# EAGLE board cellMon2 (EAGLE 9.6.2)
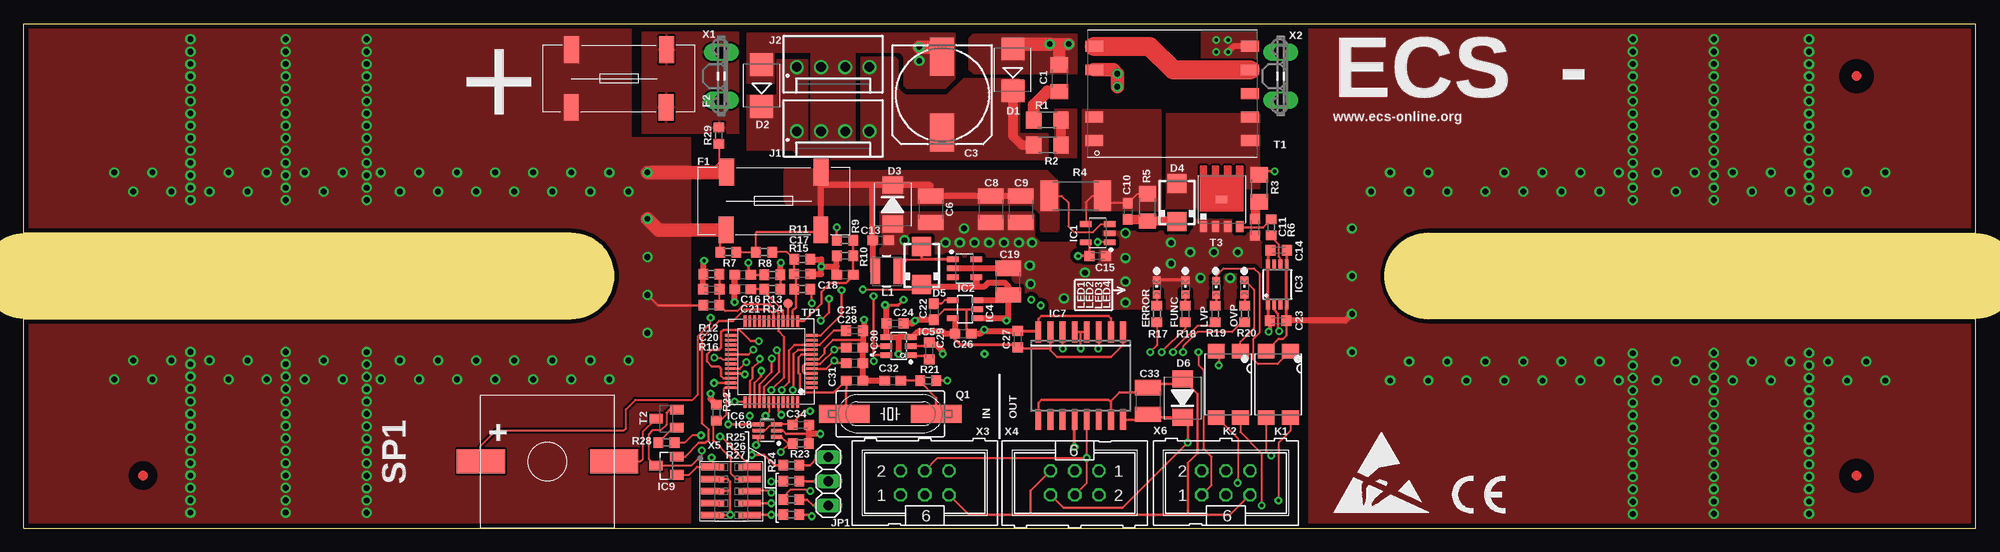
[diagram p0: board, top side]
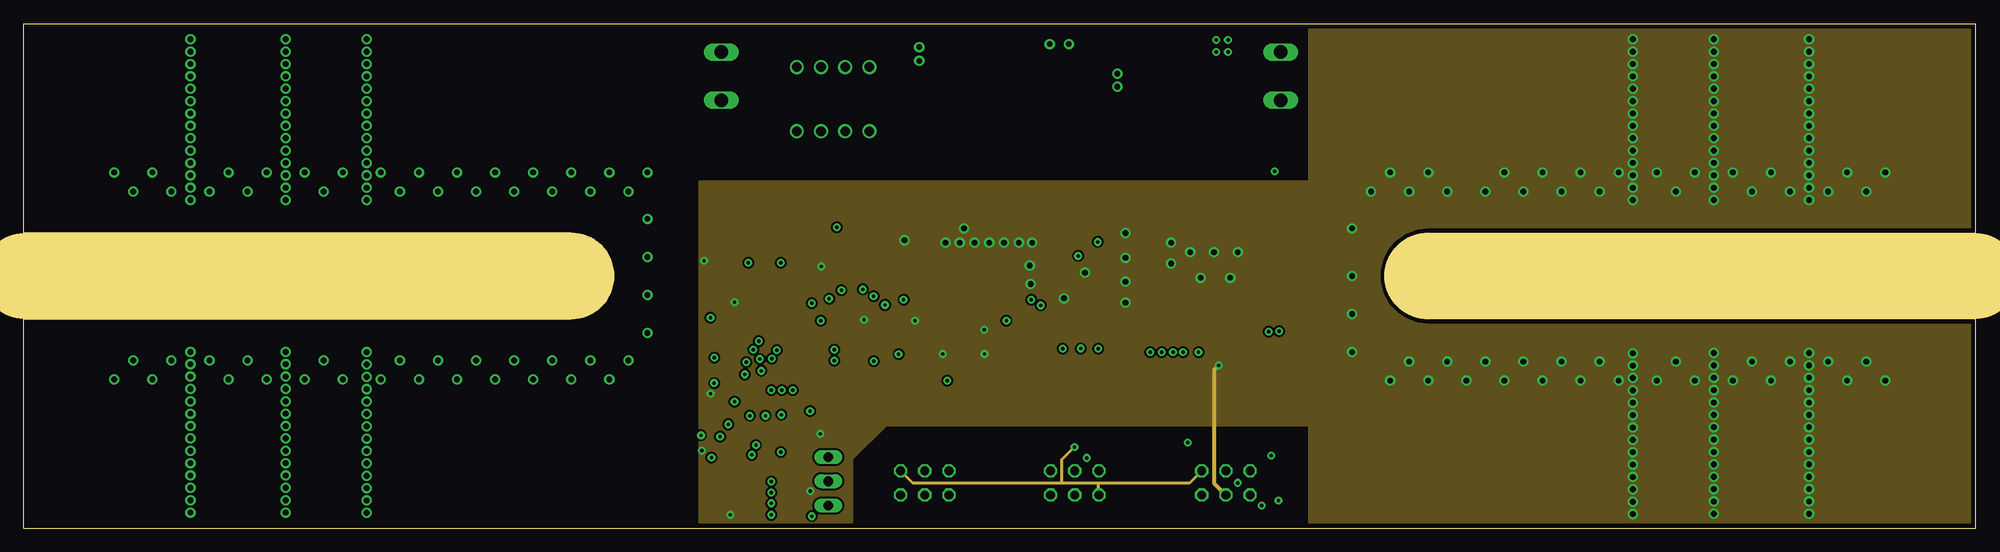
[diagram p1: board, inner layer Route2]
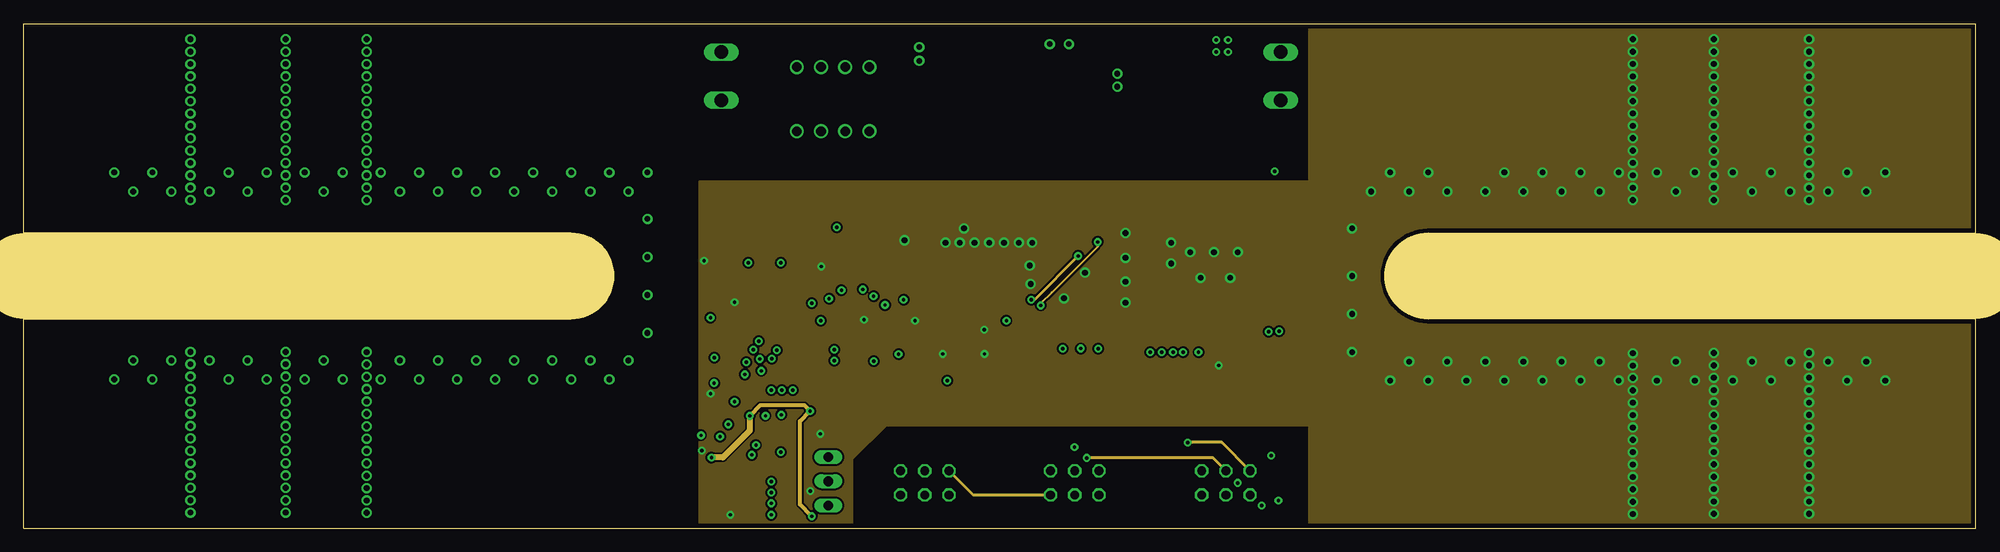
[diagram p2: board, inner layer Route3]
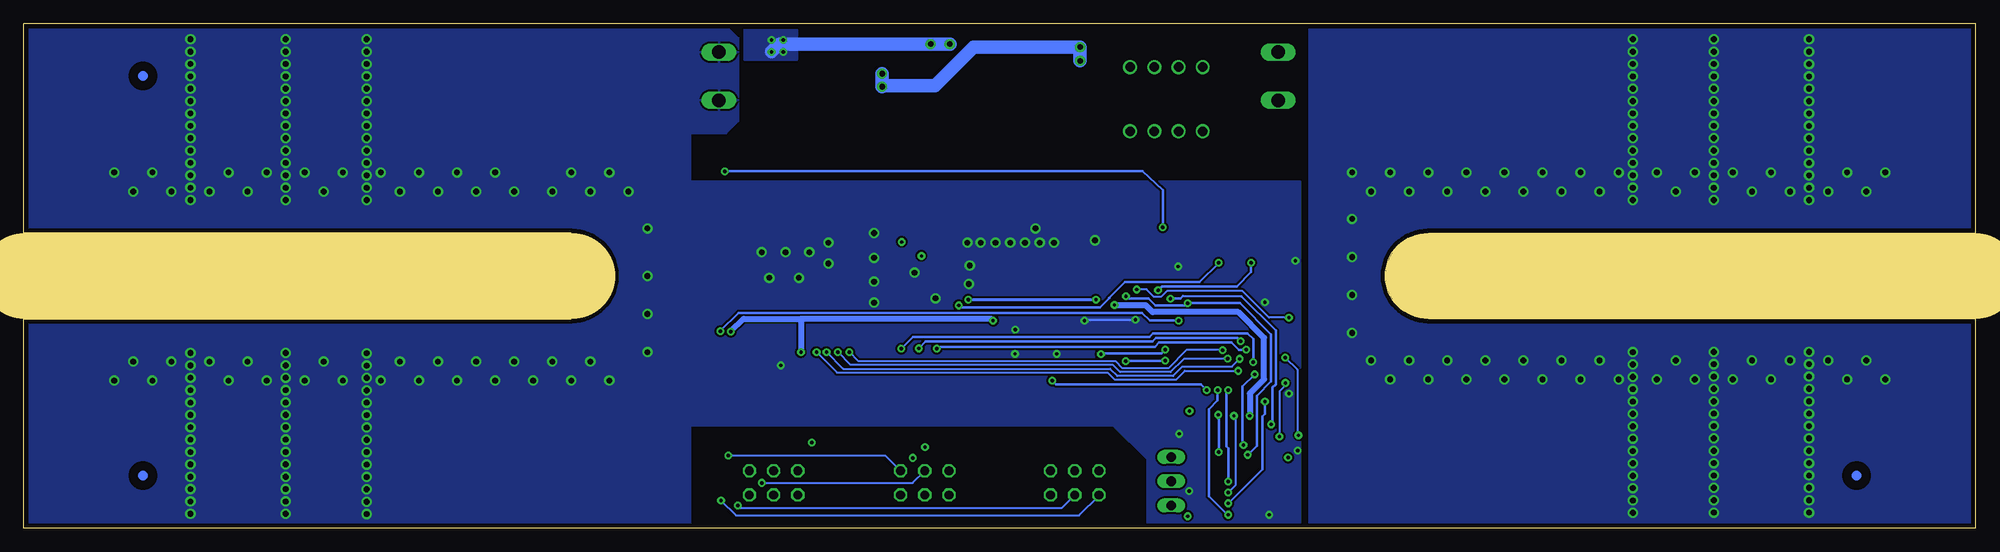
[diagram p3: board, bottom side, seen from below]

Size 205 x 53 mm. Coordinates in mm from the lower left corner, seen from the top.
Outline: 0,0 205,0 205,22 147.5,22 arc-180 147.5,31 205,31 205,53 0,53 0,31 57.5,31 arc-180 57.5,22 0,22 0,0
Copper layers (1+2*3+16): Top 0.018mm / dielectric 0.36mm / Route2 0.035mm / dielectric 0.71mm / Route3 0.035mm / dielectric 0.36mm / Bottom 0.018mm
Design rules "multi-cb_070um-cu *": minimum track width 8mil, minimum drill 12mil, track to track 8mil, track to pad 8mil, pad to pad 8mil, via to via 8mil, smd to smd 8mil, copper to edge 20mil, drill to drill 8mil, minimum pad ring 9mil, minimum via ring 9mil, stop-mask expansion 3mil, vias tented up to drill 0mil, thermal gap 8mil
Milling: 2 lines

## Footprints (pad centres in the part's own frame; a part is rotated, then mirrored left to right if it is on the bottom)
C1206 = smd 1.6 x 1.8: 1 -1.4,0; 2 1.4,0
153CLV-1010 = smd 4 x 2.5: + 4,0; - -4,0
C1210 = smd 1.6 x 2.7: 1 -1.4,0; 2 1.4,0
C0603 = smd 1.1 x 1: 1 -0.85,0; 2 0.85,0
C0603K = smd 1.05 x 1.08: 1 -0.875,0; 2 0.875,0
SMB = smd 2.4 x 2.4: A 2.2,0; C -2.2,0
SMBJ = smd 1.78 x 2.16: A 2.04,0; C -2.03,0
SMA = smd 2 x 2: A 2,0; C -2,0
3588 = smd 1.57 x 2.82: 1A -4.955,3.03; 1B -4.995,-3.03; 2A 4.995,3.03; 2B 4.955,-3.03
SOT95P280X110-5N = smd 1.209 x 0.589: 1 -1.253,0.95; 2 -1.253,0; 3 -1.253,-0.95; 4 1.253,-0.95; 5 1.253,0.95
MSOP8 = smd 0.4 x 1.2: 1 -0.975,-2.05; 2 -0.325,-2.05; 3 0.325,-2.05; 4 0.975,-2.05; 5 0.975,2.05; 6 0.325,2.05; 7 -0.325,2.05; 8 -0.975,2.05
SOT25 = smd 0.55 x 1.2: 1 -0.95,-1.3; 2 0,-1.3; 3 0.95,-1.3; 4 0.95,1.3; 5 -0.95,1.3
SOT23-6 = smd 0.55 x 1.2: 1 -0.95,-1.3; 2 0,-1.3; 3 0.95,-1.3; 4 0.95,1.3; 5 0,1.3; 6 -0.95,1.3
LQFP48 = smd 0.29 x 1.2: 1 -2.75,-4.25; 2 -2.25,-4.25; 3 -1.75,-4.25; 4 -1.25,-4.25; 5 -0.75,-4.25; 6 -0.25,-4.25; 7 0.25,-4.25; 8 0.75,-4.25; 9 1.25,-4.25; 10 1.75,-4.25; 11 2.25,-4.25; 12 2.75,-4.25; 25 2.75,4.25; 26 2.25,4.25; 27 1.75,4.25; 28 1.25,4.25; 29 0.75,4.25; 30 0.25,4.25; 31 -0.25,4.25; 32 -0.75,4.25; 33 -1.25,4.25; 34 -1.75,4.25; 35 -2.25,4.25; 36 -2.75,4.25 | smd 1.2 x 0.29: 13 4.25,-2.75; 14 4.25,-2.25; 15 4.25,-1.75; 16 4.25,-1.25; 17 4.25,-0.75; 18 4.25,-0.25; 19 4.25,0.25; 20 4.25,0.75; 21 4.25,1.25; 22 4.25,1.75; 23 4.25,2.25; 24 4.25,2.75; 37 -4.25,2.75; 38 -4.25,2.25; 39 -4.25,1.75; 40 -4.25,1.25; 41 -4.25,0.75; 42 -4.25,0.25; 43 -4.25,-0.25; 44 -4.25,-0.75; 45 -4.25,-1.25; 46 -4.25,-1.75; 47 -4.25,-2.25; 48 -4.25,-2.75
SO-16DW = smd 0.6 x 2.2: 1 -4.445,-4.6; 2 -3.175,-4.6; 3 -1.905,-4.6; 4 -0.635,-4.6; 5 0.635,-4.6; 6 1.905,-4.6; 7 3.175,-4.6; 8 4.445,-4.6; 9 4.445,4.6; 10 3.175,4.6; 11 1.905,4.6; 12 0.635,4.6; 13 -0.635,4.6; 14 -1.905,4.6; 15 -3.175,4.6; 16 -4.445,4.6
SOT65P210X110-6N = smd 1.186 x 0.397: 1 -0.962,0.65; 2 -0.962,0; 3 -0.962,-0.65; 4 0.962,-0.65; 5 0.962,0; 6 0.962,0.65
SOT23 = smd 1 x 1.4: 1 -0.95,-1.1; 2 0.95,-1.1; 3 0,1.1
61900411121 = drill 1: 1 3.81,0.3; 2 1.27,0.3; 3 -1.27,0.3; 4 -3.81,0.3
1X03 = drill 1.016 long: 1 -2.54,0; 2 0,0; 3 2.54,0
SMD4 = smd 1.78 x 1.55: 1 -1.27,-3.5; 2 1.27,-3.5; 3 1.27,3.5; 4 -1.27,3.5
WE-LQS_3015 = smd 1 x 2.7: 1 -1.2,0; 2 1.2,0
CHIPLED_0603 = smd 0.8 x 0.8: A 0,-0.75; C 0,0.75
HC49UP = smd 5.334 x 1.93: 1 -4.826,0; 2 4.826,0
R1206 = smd 1.6 x 1.803: 1 -1.422,0; 2 1.422,0
R2512 = smd 1.8 x 3.2: 1 -2.8,0; 2 2.8,0
R0603 = smd 1 x 1.1: 1 -0.85,0; 2 0.85,0
SPB45 = smd 2.54 x 5.08: P$1 0,7; P$2 0,-7
WE_EP13_SMD_9PIN = smd 1.88 x 1.143: 1 -8.18,-4.96; 2 -8.18,-2.48; 4 -8.18,2.48; 5 -8.18,4.96; 6 8.18,4.96; 7 8.18,2.48; 8 8.18,0; 9 8.18,-2.48; 10 8.18,-4.96
SOT23-BEC = smd 1 x 1.4: B -0.95,-1.1; C 0,1.1; E 0.95,-1.1
DSOP8 = smd 1.15 x 0.75: D 0,0 | smd 0.75 x 1.15: G 1.905,-2.875; S@1 -1.905,-2.875; S@2 -0.635,-2.875; S@3 0.635,-2.875
TP10R = smd 1 x 1: TP 0,0
ST6,3 = drill 1.397 long: 1 -2.54,0; 2 2.54,0
ML6 = drill 0.914 octagon: 1 -2.54,-1.27; 2 -2.54,1.27; 3 0,-1.27; 4 0,1.27; 5 2.54,-1.27; 6 2.54,1.27
PF2X5SMD50MIL = smd 0.7 x 2.4: 1 -2.54,-1.95; 2 -2.54,1.95; 3 -1.27,-1.95; 4 -1.27,1.95; 5 0,-1.95; 6 0,1.95; 7 1.27,-1.95; 8 1.27,1.95; 9 2.54,-1.95; 10 2.54,1.95

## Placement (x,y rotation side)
C1  1n0/100V  [C1206]  108.75,47.27 270 top
C3  27µ/100V/low ESR  [153CLV-1010]  96.45,45.55 270 top
C6  47uF/16V  [C1210]  95.25,33.5 270 top
C8  47uF/16V  [C1210]  101.55,33.5 270 top
C9  47uF/16V  [C1210]  104.7,33.5 270 top
C10  100n  [C0603]  115.95,33.3 270 top
C11  4n7  [C0603K]  129.3,31.6 270 top
C13  1µ  [C0603]  90,30.25 0 top
C14  100n  [C0603K]  131.8,29.2 0 top
C15  100n  [C0603K]  112.8,28.6 0 top
C16  1n  [C0603]  75.5,26.62 180 top
C17  100n  [C0603K]  81.75,26.7 0 top
C18  10p  [C0603]  86.25,26.62 180 top
C19  47uF/16V  [C1210]  103.4,25.9 90 top
C20  100n  [C0603K]  72.2,25.1 180 top
C21  1µ  [C0603]  75.5,25.12 180 top
C22  1µ  [C0603]  95.58,22.75 270 top
C23  100n  [C0603K]  131.75,21.8 0 top
C24  100n  [C0603K]  91.5,21.5 0 top
C25  100n  [C0603K]  87.25,20.75 0 top
C26  1µ  [C0603]  98.65,20.45 0 top
C27  100n  [C0603K]  104.4,19.85 90 top
C28  1µ  [C0603]  87.25,18.95 0 top
C29  100n  [C0603K]  95.1,18.62 90 top
C30  1µ  [C0603]  87.25,17.35 0 top
C31  15p  [C0603]  87.25,15.5 180 top
C32  15p  [C0603]  91.25,15.5 0 top
C33  47uF/16V  [C1210]  118.08,13.35 270 top
C34  100n  [C0603K]  81.6,10.85 0 top
D1  STPS2H100UF  [SMB]  103.88,48.15 90 top
D2  SMBJ64A  [SMB]  77.5,46.5 90 top
D3  SMBJ5A  [SMBJ]  91.25,34 270 top
D4  SS16  [SMA]  121.1,34.2 90 top
D5  SS12  [SMA]  94.3,27.6 90 top
D6  SMBJ5A  [SMBJ]  121.7,13.65 90 top
F1  3588  [3588]  78.75,34.38 0 top
F2  3588  [3588]  62.5,47.25 0 top
IC1  INA180A3QDBVRQ1  [SOT95P280X110-5N]  112.8,31 180 top
IC2  TPS613221ADBVR  [SOT95P280X110-5N]  98.8,27.3 0 top
IC3  MIC4420MM  [MSOP8]  131.65,25.6 0 top
IC4  LP2985IM5-3.3  [SOT25]  98.85,23 90 top
IC5  MAX6070BAUT25  [SOT23-6]  91.88,19.12 90 top
IC6  STM32G071CBT6TR  [LQFP48]  78.5,17.5 90 top
IC7  ADM2483BRWZ  [SO-16DW]  111,16 180 top
IC8  SN74LVC1G175DCKR  [SOT65P210X110-6N]  78.1,10.25 180 top
IC9  LM61  [SOT23]  67.47,6.55 90 top
J1  61900411121  [61900411121]  85,42 180 top
J2  61900411121  [61900411121]  85,48.75 180 top
JP1  [1X03]  84.5,4.93 270 top
K1  FOD8523S  [SMD4]  131.75,15.1 180 top
K2  FOD8523S  [SMD4]  126.5,15.1 180 top
L1  FESTINDUKTIVITÄT 10µH 0,3A 440mOhm 1210 SMD  [WE-LQS_3015]  90.62,27 0 top
LED1  rt  [CHIPLED_0603]  119,25.3 0 top
LED2  bl  [CHIPLED_0603]  122,25.3 0 top
LED3  gn  [CHIPLED_0603]  125.25,25.25 0 top
LED4  gn  [CHIPLED_0603]  128.2,25.3 0 top
Q1  Q8.000MHz/HC-49SM(SMD)/20pF  [HC49UP]  91,12 180 top
R1  47R  [R1206]  107.5,42.88 0 top
R2  47R  [R1206]  107.5,40.25 180 top
R3  4R7  [R1206]  129.75,35.7 90 top
R4  0,001/TK50  [R2512]  110.5,34.9 180 top
R5  4k7  [R1206]  118,33.7 90 top
R6  4R7  [R0603]  131,31.6 90 top
R7  10k  [R0603]  74,29 0 top
R8  18k  [R0603]  77.75,29 0 top
R9  18k  [R0603]  86.25,30.25 180 top
R10  3k  [R0603]  86.25,28.62 0 top
R11  3k  [R0603]  81.75,28.25 0 top
R12  10k/0,05%  [R0603]  72.2,26.7 180 top
R13  120R  [R0603]  78.62,26.62 0 top
R14  1k  [R0603]  78.62,25.12 0 top
R15  18k  [R0603]  81.75,25.12 180 top
R16  10k/0,05%  [R0603]  72.2,23.4 0 top
R17  4k7  [R0603]  119,22.5 90 top
R18  4k7  [R0603]  122,22.5 90 top
R19  470R  [R0603]  125.12,22.5 90 top
R20  470R  [R0603]  128.25,22.5 90 top
R21  220R  [R0603]  95,15.5 0 top
R22  100k  [R0603]  72.75,12.12 90 top
R23  18k  [R0603]  81.6,8.9 180 top
R24  1k  [R0603]  80.6,6.6 0 top
R25  10k  [R0603]  80.6,4.95 0 top
R26  10k  [R0603]  80.6,3 0 top
R27  10k  [R0603]  80.6,1.43 0 top
R28  10k  [R0603]  67.5,9 180 top
R29  10k  [R0603]  73,41.25 90 top
SP1  [SPB45]  55,7 90 top
T1  750312504  [WE_EP13_SMD_9PIN]  120.6,45.67 0 top
T2  MMBT2222  [SOT23-BEC]  67.5,11.5 90 top
T3  TPHR8504PL  [DSOP8]  125.8,34.55 0 top
TP1  TPTP10R  [TP10R]  80.25,23.62 0 top
U$1  [ESD_10.00]  137.5,1.5 0 top
U$2  [CE-4MM]  150,1.5 0 top
U$3  [CIRCLE-1MM-3R]  192.5,47.5 0 top
U$4  [CIRCLE-1MM-3R]  192.5,5.5 0 top
U$5  [CIRCLE-1MM-3R]  12.5,5.5 0 top
X1  [ST6,3]  73.25,47.5 90 top
X2  [ST6,3]  132,47.5 90 top
X3  [ML6]  94.62,4.75 0 top
X4  [ML6]  110.38,4.75 180 top
X5  JTAG  [PF2X5SMD50MIL]  74.3,3.9 270 top
X6  [ML6]  126.25,4.75 0 top

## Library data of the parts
C1 = rcl; PARTNO: C407; SPICEPREFIX: C
C3 = rcl; PARTNO: C448; SPICEPREFIX: C
C6 C8 C9 C19 C33 = rcl; PARTNO: C219; SPICEPREFIX: C
C10 = rcl; PARTNO: C059; SPICEPREFIX: C
C11 = rcl; PARTNO: C051; SPICEPREFIX: C
C13 C21 C22 C26 C28 C30 = rcl; PARTNO: C079; SPICEPREFIX: C
C14 C15 C17 C20 C23-C25 C27 C29 C34 = rcl; PARTNO: C067; SPICEPREFIX: C
C16 = rcl; PARTNO: C043; SPICEPREFIX: C
C18 = rcl; PARTNO: C427; SPICEPREFIX: C
C31 C32 = resistor; PARTNO: C249
D1 = diode; PARTNO: D093
D2 = diode; PARTNO: D203
D3 D6 = diode; PARTNO: D087
D4 = diode; PARTNO: D089
D5 = diode; DNP: T; PARTNO: D090
F1 = fuse_keystone_3568; PARTNO: EM011
F2 = fuse_keystone_3568; DNP: T; PARTNO: EM011
IC1 = ina180; PARTNO: IC325
IC2 = TPS613221; PARTNO: IC328
IC3 = my_transistor-power; PARTNO: IC039
IC4 = v-reg; PARTNO: IC026
IC5 = max6070; PARTNO: IC326
IC6 = STM32G070CB; PARTNO: IC321
IC7 = texas; MPN: ISO1176DW; OC_FARNELL: 1755037; OC_NEWARK: 13N4111; PARTNO: IC002
IC8 = 74LVC1G175; PARTNO: IC329
IC9 = linear; PARTNO: IC040
J1 J2 = Wurth_Connectors_WR-WTB; CONTACT-RESISTANCE: 20mOhm; DATASHEET-URL: https://www.we-online.com/redexpert/spec/61900411121?ae; GENDER: Male; L: 10.16mm; MOUNT: THT; PACKAGING: Bag; PART-NUMBER: 61900411121; PCB-CABLE-PANEL: PCB; PINS: 4; PITCH: 2.54mm; TYPE: Vertical; WORKING-VOLTAGE: 250V(AC)
JP1 = pinhead; PARTNO: CON031
K1 K2 = optocoupler; OC_FARNELL: unknown; OC_NEWARK: unknown; PARTNO: IC053
L1 = Wurth_Power Magnetics_WE-LQS; DATASHEET-URL: https://www.we-online.com/catalog/datasheet/74404032022.pdf; FRES: 75MHz; IR: 1.8A; ISAT: 1.7A; PART-NUMBER: 74404032022; PARTNO: L114; RDC: 50mOhm
LED1 = led; PARTNO: D079
LED2 = led; PARTNO: D077
LED3 LED4 = led; PARTNO: D078
Q1 = crystal; OC_FARNELL: unknown; OC_NEWARK: unknown; PARTNO: Q003
R1 R2 = rcl; PARTNO: R574; SPICEPREFIX: R
R3 = rcl; PARTNO: R550; SPICEPREFIX: R
R4 = rcl; PARTNO: R826; SPICEPREFIX: R
R5 = rcl; PARTNO: R622; SPICEPREFIX: R
R6 = rcl; PARTNO: R141; SPICEPREFIX: R
R7 R25-R28 = rcl; PARTNO: R221; SPICEPREFIX: R
R8 R9 R15 R23 = rcl; PARTNO: R227; SPICEPREFIX: R
R10 R11 = rcl; PARTNO: R208; SPICEPREFIX: R
R12 R16 = rcl; PARTNO: R869; SPICEPREFIX: R
R13 = rcl; PARTNO: R175; SPICEPREFIX: R
R14 = rcl; PARTNO: R197; SPICEPREFIX: R
R17 R18 = rcl; PARTNO: R213; SPICEPREFIX: R
R19 R20 = rcl; PARTNO: R189; SPICEPREFIX: R
R21 = resistor; PARTNO: R181
R22 = resistor; PARTNO: R245
R24 = rcl; SPICEPREFIX: R
R29 = rcl; DNP: T; PARTNO: R221; SPICEPREFIX: R
SP1 = mBuzzer
T1 = Wuerth_Elektronik_eiSos_V6; PARTNO: L096
T2 = transistor
T3 = TPW_MOSFET; PARTNO: T134
TP1 = testpad
U$1 U$2 = logo
U$3-U$5 = fidu
X1 X2 = con-rib; DNP: T; OC_FARNELL: unknown; OC_NEWARK: unknown
X3 X4 = con-harting-ml; OC_FARNELL: unknown; OC_NEWARK: unknown; PARTNO: CON207
X5 = A_CONN; PARTNO: CON156
X6 = con-harting-ml; DNP: T; OC_FARNELL: unknown; OC_NEWARK: unknown; PARTNO: CON207

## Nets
+: C1.1 D1.A T1.6
+5V: C14.1 C19.1 C23.1 D5.C IC2.4 IC3.1 IC3.8 IC4.1 IC4.3 SP1.P$1 X6.1
+UB: F1.1A F1.1B F2.1A F2.1B R7.1 R16.1 R29.1
A: IC7.12 X3.2 X4.2 X6.2
ADC1_IN5_I_SENSE_AVG: C21.1 IC6.16 R14.1
ADC1_IN6_UIN_SENSE: C20.1 IC6.17 R12.1 R16.2 R25.1
ADC1_IN6_UIN_SENSE_: JP1.2 R25.2
ADC1_IN7_TEMP_SENSE: IC6.18 IC9.2
B: IC7.13 X3.4 X4.4 X6.4
COMP1_INP_I_SENSE: C16.1 IC6.12 R13.1
COMP1_OUT_I_PEAK: IC6.33 IC8.6
COMP2_INM_U_TR_SENSE: C18.1 IC6.13 R9.1 R10.2
COMP2_INP_U_TR_REF: C17.1 IC6.14 R8.2 R11.1 R15.2
COMP2_OUT_DISCHARGE: IC6.44 IC8.1 R23.2
DAC1_OUT1_I_CTR_TP: IC6.15 TP1.TP
GND: C6.2 C8.2 C9.2 C11.2 C13.2 C14.2 C15.2 C16.2 C17.2 C18.2 C19.2 C20.2 C21.2 C22.2 C23.2 C24.2 C25.2 C26.2 C27.2 C28.2 C29.2 C30.2 C31.1 C32.1 C34.2 D3.A IC1.2 IC2.2 IC3.4 IC3.5 IC4.2 IC5.2 IC6.7 IC7.2 IC7.8 IC8.2 IC9.3 K1.2 K2.2 LED1.C LED2.C R10.1 R11.2 R12.2 R22.2 R23.1 R26.1 T2.E T3.S@1 T3.S@2 T3.S@3 X2.1 X2.2 X5.3 X5.5 X5.9 X6.3
GND2: C33.1 D6.A IC7.9 IC7.15 X3.5 X4.5 X6.5
IS-: C10.1 IC1.4 R4.1 R5.2 T1.1 T1.2
LED_ERROR: IC6.41 R17.1
LED_FUNC: IC6.40 R18.1
LPUART1_DE: IC6.34 IC7.4 IC7.5
LPUART1_RX: IC6.32 IC7.3
LPUART1_TX: IC6.29 IC7.6
LVP: IC6.38 R19.1
LVP_IN: K1.4 X3.1
LVP_OUT: K1.3 X4.1
N$1: IC3.6 R6.1
N$2: R1.2 R2.1
N$3: C31.2 IC6.8 Q1.2
N$4: D5.A IC2.1 L1.2
N$5: C1.2 R1.1
N$6: C22.1 IC4.4
N$7: C3.- D2.A J1.2 J1.3 J2.2 J2.3 T1.4
N$8: IC3.2 IC8.4
N$9: IC6.9 R21.2
N$10: SP1.P$2 T2.C
N$11: T1.5 T1.7
N$12: C32.2 Q1.1 R21.1
N$14: IC1.1 R13.2 R14.2
N$16: R28.2 T2.B
N$17: C3.+ D1.C D2.C J1.1 J1.4 J2.1 J2.4 R2.2
N$18: LED4.A R20.2
N$19: LED3.A R19.2
N$20: R6.2 T3.G
N$21: JP1.3 R26.2
N$22: C29.1 IC5.1
N$23: C11.1 R3.1
N$24: D4.A R3.2 R9.2 T1.9 T1.10 T3.D
N$25: C10.2 D4.C R5.1
N$26: IC6.30 R28.1
N$28: F2.2A F2.2B R29.2 X1.1 X1.2
N$31: LED2.A R18.2
N$34: LED1.A R17.2
N$35: K2.1 LED4.C
N$36: K1.1 LED3.C
NRST: C25.1 IC6.10 R27.1 X5.10
OVP: IC6.39 R20.1
OVP_IN: K2.4 X3.3
OVP_OUT: K2.3 X4.3
R1: IC6.42 X5.6
R2: IC6.37 X5.8
SWCLK: IC6.36 R22.1 X5.4
SWDIO: IC6.35 X5.2
VCC: C15.1 C24.1 C26.1 C27.1 C28.1 C34.1 IC1.5 IC4.5 IC5.3 IC5.4 IC6.4 IC6.6 IC7.1 IC7.7 IC8.3 IC8.5 IC9.1 R27.2 X5.1
VCC2: C33.2 D6.C IC7.16 X3.6 X4.6 X6.6
VIN: C6.1 C8.1 C9.1 C13.1 D3.C F1.2A F1.2B IC1.3 L1.1 R4.2 R7.2 R8.1
VREF: C30.1 IC5.5 IC5.6 IC6.5 R15.1 R24.1
VREF_: JP1.1 R24.2

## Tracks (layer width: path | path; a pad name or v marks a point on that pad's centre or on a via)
+  (via drill 0.35, 0.6)
  Top 0.61: v126.47,50.05 127.06,50.64 T1.6
  Top 1.27: v107.75,50.88 v109.75,50.88 108.75,50.88 C1.1
  Top 1.422: D1.A 104.4,50.88 v107.75,50.88
  Bottom 1.422: v126.47,50.05 125.65,50.88 v107.75,50.88
  other vias: 126.47,51.3 125.22,51.3 125.22,50.05
  pour Top (no thermals): 99.75,51.89 110.55,51.89 110.55,47.75 99.8,47.75 99.35,48.2 99.35,51.48
  pour Top (no thermals): 123.75,52.12 129.38,52.12 129.38,49.25 123.75,49.25
  pour Bottom: 123.75,52.38 129.38,52.38 129.38,49.25 123.75,49.25
+5V  (via drill 0.35)
  Top 0.203: X6.1 124.75,4.52 124.75,7.5 123.88,8.38 123.88,16.62 123.38,17.12 v123.38,18.5 | SP1.P$1 48,8.62 49.62,10.25 63,10.25 63.25,10.5 63.25,12.5 64.25,13.5 70.25,13.5 70.81,14.06 70.81,20.17 72.12,21.49 v72.12,22.12 | v88.12,25.08 93.78,25.08 D5.C
  Top 0.305: C23.1 130.68,22 IC3.1 IC3.8 130.68,28.95 C14.1
  Top 0.406: C23.1 130.88,20.77 v130.75,20.65
  Top 0.61: D5.C 94.5,25.4 100.1,25.4 | C19.1 103.4,25.4 103,25.8 101.3,25.8 100.9,25.4 100.1,25.4 | IC4.3 102.85,23.95 C19.1 | IC4.1 102.95,22.05 v103.2,21.8 103.4,22 C19.1 | IC2.4 100.05,25.45 100.1,25.4
  Bottom 0.203: v72.12,22.12 74.21,22.12 77,24.92 84.96,24.92 85.58,24.29 86.29,24.29 87.08,25.08 v88.12,25.08
  Bottom 0.61: v130.75,20.65 129.4,22 123.38,22 | 123.38,22 v123.38,18.5 | v103.2,21.8 103.4,22 123.38,22
+UB  (via drill 0.6)
  Top 0.203: R29.1 73,38.36 72.02,37.38
  Top 0.254: F1.1B 73.15,30.74 R7.1 | R16.1 66.6,23.4 v65.5,24.5
  Top 1.422: v65.5,37.38 72.02,37.38 73.77,37.38 F1.1A | v65.5,32.5 66.66,31.34 F1.1B
  other vias: 37.5,37.38 39.5,35.38 41.5,37.38 43.5,35.38 47.5,35.38 49.5,37.38 51.5,35.38 53.5,37.38 29.5,37.38 33.5,37.38 31.5,35.38 45.5,37.38 55.5,35.38 57.5,37.38 27.5,51.38 27.5,50.08 27.5,48.77 27.5,47.48 27.5,46.17 27.5,44.88 27.5,43.58 27.5,42.27 27.5,40.98 27.5,39.67 27.5,38.38 27.5,37.08 27.5,35.77 27.5,34.48 15.5,35.38 19.5,35.38 21.5,37.38 23.5,35.38 9.5,37.38 13.5,37.38 11.5,35.38 25.5,37.38 27.5,18.52 27.5,17.23 27.5,15.93 27.5,14.62 27.5,13.32 27.5,12.03 27.5,10.72 27.5,9.43 27.5,8.12 27.5,6.82 27.5,5.52 27.5,4.23 27.5,2.93 27.5,1.62 19.5,17.62 15.5,17.62 13.5,15.62 11.5,17.62 25.5,15.62 21.5,15.62 23.5,17.62 9.5,15.62 51.5,17.62 49.5,15.62 47.5,17.62 45.5,15.62 43.5,17.62 39.5,17.62 37.5,15.62 33.5,15.62 57.5,15.62 53.5,15.62 55.5,17.62 41.5,15.62 31.5,17.62 29.5,15.62 59.5,17.62 61.5,15.62 63.5,17.62 65.5,20.5 59.5,35.38 63.5,35.38 61.5,37.38 65.5,28.5 17.5,51.38 17.5,50.08 17.5,48.77 17.5,47.48 17.5,46.17 17.5,44.88 17.5,43.58 17.5,42.27 17.5,40.98 17.5,39.67 17.5,38.38 17.5,37.08 17.5,35.77 17.5,34.48 17.5,18.52 17.5,17.23 17.5,15.93 17.5,14.62 17.5,13.32 17.5,12.03 17.5,10.72 17.5,9.43 17.5,8.12 17.5,6.82 17.5,5.52 17.5,4.23 17.5,2.93 17.5,1.62 36,18.5 36,17.2 36,15.9 36,14.6 36,13.3 36,12 36,10.7 36,9.4 36,8.1 36,6.8 36,5.5 36,4.2 36,2.9 36,1.6 36,51.38 36,50.08 36,48.77 36,47.48 36,46.17 36,44.88 36,43.58 36,42.27 36,40.98 36,39.67 36,38.38 36,37.08 36,35.77 36,34.48
  pour Top (no thermals): 70,0 70,41 63.75,41 63.75,53 0,53 0,0
  pour Bottom (no thermals): 70,53 0,53 0,0 70,0
A  (via drill 0.35)
  Top 0.305: v110.35,8.52 110.35,11.38 IC7.12
  Route2 0.305: X6.2 122.42,4.73 112.88,4.73 | 112.88,4.73 109,4.73 | 109,4.73 93.38,4.73 X3.2 | X4.2 112.88,3.52 112.88,4.73 | v110.35,8.52 109,7.18 109,4.73
ADC1_IN5_I_SENSE_AVG
  Top 0.254: IC6.16 79.75,22.86 77.75,24.86 R14.1 C21.1
ADC1_IN6_UIN_SENSE  (via drill 0.35)
  Top 0.203: 78.36,23.52 75.66,23.52 74.94,22.8 73.69,22.8 73.08,23.43 | R16.2 73.05,25.07 C20.1
  Top 0.254: v78.5,14.5 79.85,15.85 79.85,20.1 79.25,20.7 IC6.17 79.25,22.63 78.36,23.52 | R25.1 79.7,4.9 v78.5,4.9 | R12.1 73.05,25.12 C20.1 | 73.08,23.43 R16.2
  Bottom 0.254: v78.5,14.5 78.7,14.3 78.7,8.6 78.5,8.4 v78.5,4.9
ADC1_IN6_UIN_SENSE_
  Top 0.254: JP1.2 81.47,4.93 R25.2
ADC1_IN7_TEMP_SENSE
  Top 0.254: IC6.18 78.75,22.48 78.28,22.95 75.7,22.95 74.5,21.75 73,21.75 71.24,19.99 71.25,11.03 71.9,10.36 71.9,9.28 71.58,8.95 70.88,8.95 69.42,7.5 IC9.2
B  (via drill 0.35)
  Top 0.203: IC7.13 v111.62,7.38 | X3.4 95.98,7.38 v111.62,7.38 | v111.62,7.38 111.62,4.73 X4.4
  Route3 0.305: X6.4 124.89,7.38 v111.62,7.38
COMP1_INP_I_SENSE  (via drill 0.35)
  Top 0.254: IC6.12 83.67,20.25 85.88,22.45 v85.88,25 | R13.1 C16.1 76.1,26.7 v76.1,27.9
  Bottom 0.254: v85.88,25 85.47,25.4 77.6,25.4 76.1,26.9 v76.1,27.9
COMP1_OUT_I_PEAK  (via drill 0.35)
  Top 0.254: v76.9,8.71 77.14,8.95 IC8.6 | v75.72,16.15 75.62,16.25 IC6.33
  Bottom 0.254: v75.72,16.15 77,14.88 77,8.81 v76.9,8.71
COMP2_INM_U_TR_SENSE
  Top 0.254: IC6.13 81.95,21.75 83.8,23.6 83.8,24.8 84.75,25.75 86.35,25.75 86.5,25.9 C18.1 R10.2 R9.1
COMP2_INP_U_TR_REF
  Top 0.203: R11.1 80.15,29 R8.2
  Top 0.254: IC6.14 80.75,22.85 81.1,23.2 81.1,24.9 | 81.1,24.9 R15.2 | R11.1 80.9,26.73 C17.1 81.1,26.48 81.1,24.9
COMP2_OUT_DISCHARGE  (via drill 0.35)
  Top 0.203: R23.2 80.25,8.9 79.65,9.5 79.16,9.5 IC8.1
  Top 0.254: IC6.44 79.25,12.25 79.56,11.94 v79.56,11.91 | R23.2 80.4,8.9 v79.5,8
  Bottom 0.254: v79.56,11.91 79.5,11.85 v79.5,8
DAC1_OUT1_I_CTR_TP
  Top 0.254: IC6.15 TP1.TP
GND  (via drill 0.35, 0.6)
  Top 0.203: v71.2,8.15 71.2,7.65 70.1,6.55 IC9.3 65.62,7.3 65.62,9.88 66,10.25 66.88,10.25 67.5,10.88 67.5,12.12 67.83,12.45 T2.E | R26.1 79.75,3.25 80.5,4 82.5,4 v82.6,3.9 | K2.2 125.5,18.33 v125.5,17.1
  Top 0.254: IC5.2 94.72,19.12 C29.2 | C26.2 99,20.95 99,23 | IC4.2 99,23 | IC6.7 83.48,17.75 84.08,18.35 84.08,18.91 84.97,19.8 88.03,19.8 88.12,19.7 | 99,23 96.67,23 C22.2 | IC7.2 114.17,22.02 113.9,22.3 106.9,22.3 106.56,21.95 106.56,20.7 IC7.8 | IC8.2 79.69,10.25 80.06,9.88 82.23,9.88 82.45,10.1 | 74.2,3.9 v74.2,1.4 74.16,1.36 X5.9 | 74.2,3.9 74.2,4.9 73.93,5.17 X5.3 | X5.5 74.2,3.9 | K1.2 131.75,19.88 132.25,19.88 132.62,20.25 C23.2
  Top 0.305: C27.2 106.53,20.73 106.56,20.7 | C23.2 IC3.4 IC3.5 132.62,29.15 C14.2 | LED2.C LED1.C
  Top 0.61: C32.1 C31.1 C30.2 C28.2 88.12,18.98 88.12,19.7 C25.2 88.25,20.88 v88.25,21.9 | v74.65,23.75 C16.2 C21.2 | C24.2 93.3,21.5 v93.6,21.8 93.7,21.9 C22.2 | v96.5,18.3 96.5,18.6 95.8,19.3 95.3,19.3 C29.2 | C19.2 IC2.2 | v139.5,22.5 138.8,21.8 C23.2 | C20.2 71.33,26.68 R12.2 71.35,28 v71.45,28.1 | C18.2 85.38,27.5 | 85.38,27.5 R10.1 | v83.75,27.5 85.38,27.5 | C26.2 100.47,20.45 v100.88,20.85 101,20.73 C27.2 | R23.1 82.45,9.9 | 82.45,9.9 82.45,10.1 82.45,10.82 C34.2 | v83.65,9.9 82.45,9.9 | v72.12,14.12 72.12,13.6 R22.2 | R11.2 83.75,28.25 v83.75,27.5 | C17.2 83.75,26.7 v83.75,27.5
  Route2 0.406: v125.5,17.1 125,16.6 125,4.73 X6.3
  Bottom 0.254: v93.6,21.8 93.5,21.9 v88.25,21.9
  other vias: 139.5,31.5 139.5,26.5 139.5,18.5 177.5,51.38 177.5,50.08 177.5,48.77 177.5,47.48 177.5,46.17 177.5,44.88 177.5,43.58 177.5,42.27 177.5,40.98 177.5,39.67 177.5,38.38 177.5,37.08 177.5,35.77 177.5,34.48 177.5,1.5 177.5,2.8 177.5,4.1 177.5,5.4 177.5,6.7 177.5,8 177.5,9.3 177.5,10.6 177.5,11.9 177.5,13.2 177.5,14.5 177.5,15.8 177.5,17.1 177.5,18.4 195.5,37.38 193.5,35.38 191.5,37.38 189.5,35.38 185.5,35.38 183.5,37.38 181.5,35.38 179.5,37.38 175.5,37.38 173.5,35.38 171.5,37.38 167.5,37.38 165.5,35.38 163.5,37.38 161.5,35.38 159.5,37.38 157.5,35.38 155.5,37.38 153.5,35.38 175.5,15.5 173.5,17.5 171.5,15.5 167.5,15.5 165.5,17.5 163.5,15.5 161.5,17.5 159.5,15.5 157.5,17.5 155.5,15.5 153.5,17.5 151.5,15.5 179.5,15.5 181.5,17.5 183.5,15.5 185.5,17.5 189.5,17.5 191.5,15.5 193.5,17.5 195.5,15.5 149.5,17.5 147.5,15.5 145.5,17.5 143.5,15.5 149.5,35.38 147.5,37.38 145.5,35.38 143.5,37.38 141.5,35.38 100.9,18.3 187.5,51.38 187.5,50.08 187.5,48.77 187.5,47.48 187.5,46.17 187.5,44.88 187.5,43.58 187.5,42.27 187.5,40.98 187.5,39.67 187.5,38.38 187.5,37.08 187.5,35.77 187.5,34.48 187.5,1.5 187.5,2.8 187.5,4.1 187.5,5.4 187.5,6.7 187.5,8 187.5,9.3 187.5,10.6 187.5,11.9 187.5,13.2 187.5,14.5 187.5,15.8 187.5,17.1 187.5,18.4 122.5,29 125,29 126.7,26.3 123.6,26.3 115.7,23.7 120.5,30 120.5,27.8 115.7,28.4 115.7,31 105.9,30 102.95,30 99.85,30 96.8,30 98.75,31.5 92.5,30.25 98.3,30 101.4,30 104.5,30 105.65,27.6 105.75,25.65 111.45,26.85 115.7,25.9 109.25,24.15 127.5,29 169,51.38 169,50.08 169,48.77 169,47.48 169,46.17 169,44.88 169,43.58 169,42.27 169,40.98 169,39.67 169,38.38 169,37.08 169,35.77 169,34.48 169,18.38 169,17.07 169,15.78 169,14.47 169,13.18 169,11.88 169,10.57 169,9.27 169,7.98 169,6.68 169,5.38 169,4.07 169,2.77 169,1.48
  pour Bottom: 70.95,0 70.95,36.4 135,36.4 135,41.5 131.25,41.5 130,42.75 130,51.5 131.5,53 205,53 205,0 135,0 135,10.8 90.6,10.8 87,7.2 87,0
  pour Top (isolate 0.305): 205,53 135,53 135,0 205,0
  pour Top (isolate 0.406, no thermals): 88.17,30.9 88.17,32.8 88.58,33.2 105.8,33.2 106.1,32.9 106.1,30.7 106.8,30 113.05,30 113.4,30.35 113.4,31.2 113.45,31.15 122.55,31.15 122.95,31.55 122.95,32.5 123,32.45 127.05,32.45 128,31.5 128.5,31.5 129.95,30.05 129.95,25.95 129.5,25.5 129.45,25.5 127,23.05 105.06,23.05 103.9,24.21 103.9,27.1 102.5,28.5 88.2,28.5
  pour Route2: 87,0 70.95,0 70.95,36.4 135,36.4 135,53 205,53 205,0 135,0 135,10.8 90.6,10.8 87,7.2
  pour Route3: 87,0 70.95,0 70.95,36.4 135,36.4 135,53.05 205,53.05 205,0 135,0 135,10.8 90.6,10.8 87,7.2
GND2
  Top 0.254: X6.5 126.69,1.38 122.25,1.38 | 122.25,1.38 105.75,1.38 | 105.75,1.38 99.27,1.38 X3.5 | X4.5 105.75,3.93 105.75,1.38 | 122.25,1.38 122.25,6.88 123.25,7.88 123.25,14.12 121.7,15.68 D6.A 121.16,15.15 118.47,15.15 C33.1 117.58,14.25 115.05,14.25 114.17,13.38 114.17,13.25 | IC7.15 114.17,13.25 | IC7.9 106.56,13.18 106.88,13.5 113.92,13.5 114.17,13.25
IS-
  Top 0.203: IC1.4 111.55,34.25 112.2,34.9 R4.1 114.05,34.15 C10.1 116.92,35.12 R5.2
  pour Top (no thermals): 111.25,44 119.38,44 119.38,33.38 111.25,33.38
LED_ERROR  (via drill 0.35)
  Top 0.203: R17.1 119,19.2 v118.3,18.5
  Top 0.254: v79.1,18.7 79.3,18.5 79.3,16.4 77.75,14.85 IC6.41
  Bottom 0.203: v79.1,18.7 82.9,18.7 84.8,16.8 89.6,16.8 90.37,17.57 117.37,17.57 v118.3,18.5
LED_FUNC  (via drill 0.35)
  Top 0.203: R18.1 122,21 v119.5,18.5
  Top 0.254: v78.55,17.8 78.55,16.4 77.25,15.1 IC6.40
  Bottom 0.203: v78.55,17.8 83.15,17.8 84.56,16.39 89.87,16.39 90.64,17.16 118.16,17.16 v119.5,18.5
LPUART1_DE  (via drill 0.35)
  Top 0.254: IC7.5 111,20.6 | 111,20.6 IC7.4 | v111,18.88 111,20.6 | v77.2,19.65 76.35,19.65 75.15,20.85 73.47,20.85 73.22,20.6 73.22,19 73,18.75 72.25,18.75 71.75,18.25 71.75,17.5 72.25,17 73,17 73.25,16.75 73.25,16 73.5,15.75 IC6.34
  Bottom 0.254: v111,18.88 110.28,19.6 86.47,19.6 86.08,20 77.55,20 v77.2,19.65
LPUART1_RX  (via drill 0.35)
  Top 0.254: v112.85,18.85 112.91,18.91 IC7.3 | IC6.32 75.17,16.75 v75.88,17.45
  Bottom 0.254: v112.85,18.85 111.6,20.1 86.8,20.1 86.43,20.47 76.47,20.47 75.88,19.88 v75.88,17.45
LPUART1_TX  (via drill 0.35)
  Top 0.254: IC7.6 v109.1,18.85 | IC6.29 76.12,18.25 v76.62,18.75
  Bottom 0.254: v109.1,18.85 108.9,19.05 86.21,19.05 85.76,19.5 78.15,19.5 77.4,18.75 v76.62,18.75
LVP  (via drill 0.35)
  Top 0.203: R19.1 124.72,21.25 123.25,21.25 120.7,18.7 v120.7,18.5
  Top 0.254: IC6.38 76.25,15.45 76.55,15.75 76.55,16.82 77.3,17.57 v77.3,17.77
  Bottom 0.203: v77.3,17.77 78.1,16.98 83.3,16.98 84.29,15.99 90.14,15.99 90.9,16.75 118.95,16.75 v120.7,18.5
LVP_IN  (via drill 0.35)
  Top 0.203: K1.4 133.02,10.23 131.77,8.98 v131.77,2.89
  Bottom 0.203: v131.77,2.89 130.22,1.34 94.16,1.34 92.09,3.41 X3.1
LVP_OUT  (via drill 0.35)
  Top 0.203: K1.3 130.48,8.14 v131,7.62
  Bottom 0.203: v131,7.62 130.98,7.64 114.54,7.64 X4.1
N$1
  Top 0.203: IC3.6 131.97,28.35 131.83,28.5 131.83,29.79 131,30.62 R6.1
N$2
  Top 1.016: R1.2 R2.1
  pour Top (no thermals): 108.35,44.02 110.53,44.02 110.53,38.95 108.35,38.95
N$3
  Top 0.254: IC6.8 81.7,18.25 81.36,17.91 81.36,16.28 81.5,16.14 81.5,14.5 81.75,14.25 85.05,14.25 C31.2 86.3,12.13 Q1.2
N$4
  Top 0.203: L1.2 92.75,28.25 94.3,28.25
  Top 0.305: IC2.1 94.3,28.25 D5.A
N$5
  Top 1.27: C1.2 107.5,45.88 106.08,44.45 R1.1
N$6
  Top 0.254: IC4.4 96.75,23.95 96.4,23.6 C22.1
N$7  (via drill 0.6)
  Top 1.422: C3.- 95.45,50.55 v94.05,50.55 | v114.85,46.4 v114.85,47.75 114.44,48.16 T1.4
  Bottom 1.422: v114.85,46.4 v114.85,47.75 114.85,46.5 109.33,46.5 105.28,50.55 v94.05,50.55 v94.05,49.1
  pour Top (no thermals): 97.75,52 97.75,47.25 96.75,46.25 92.75,46.25 92.5,46.5 92.5,49.5 92,50 87.25,50 87.25,40.75 82.75,40.75 82.75,50 78.75,50 78.75,46.75 76,46.75 76,51.99
N$8  (via drill 0.35)
  Top 0.254: IC8.4 v74,10.9 | v84.58,24.11 84.58,22.66 v83.7,21.79 | v131.85,20.7 131.73,20.82 131.73,22.5 131.32,22.9 IC3.2
  Bottom 0.254: v74,10.9 73.85,11.05 73.85,14.78 73.51,15.12 73.5,20.75 77.11,24.36 83.25,24.38 83.52,24.11 v84.58,24.11 | v83.7,21.79 83.71,21.8 86.71,21.8 87.55,22.63 129.92,22.63 v131.85,20.7
N$9  (via drill 0.35)
  Top 0.254: IC6.9 81.3,18.75 80.85,18.3 80.85,14.6 v80.75,14.5 | R21.2 v97,15.5
  Bottom 0.254: v97,15.5 96.6,15.1 81.35,15.1 v80.75,14.5
N$10
  Top 0.203: T2.C 65,10.1 65,7.25 64.75,7 SP1.P$2
N$11
  Top 2: T1.7 120.72,48.16 118.24,50.64 T1.5
N$12
  Top 0.254: R21.1 94,15.5 | 94,15.5 C32.2 | Q1.1 95.83,13.67 94,15.5
N$14  (via drill 0.35)
  Top 0.203: v112.8,30.07 112.82,30.05 IC1.1
  Top 0.254: R13.2 R14.2
  Top 0.61: R13.2 79.47,27.88 v79.5,27.88
  Route3 0.203: v112.8,30.07 112.8,29.6 107.97,24.77 | 107.97,24.77 106.8,23.6 v106.8,23.4 | 107.97,24.77
  Bottom 0.254: v79.5,27.88 81.54,25.86 89.36,25.86 91,24.21 90.99,24.21 92,23.2 106.6,23.2 v106.8,23.4
N$16
  Top 0.203: R28.2 68.2,10.55 T2.B
N$17
  Top 1.016: R2.2 104.83,40.25 103.88,41.2 D1.C
  pour Top (no thermals): 107.5,41.45 107.5,38.75 84,38.75 83.5,39.25 81.25,39.25 80.77,39.73 76,39.73 76,45.51 79.18,45.51 79.18,49.25 82.25,49.25 82.25,40.25 88,40.25 88,49.5 91.5,49.5 91.75,49.25 91.75,46.25 92.5,45.5 96.97,45.5 98.76,47.25 104.5,47.25 104.5,41.38 104.58,41.45
N$18
  Top 0.254: LED4.A 128.25,24.5 R20.2
N$19
  Top 0.254: LED3.A 125.25,23.48 R19.2
N$20
  Top 0.254: R6.2 130.15,31.6 127.78,31.6 T3.G
N$21
  Top 0.254: JP1.3 82.86,2.39 82.25,3 R26.2
N$22
  Top 0.254: IC5.1 93.28,18.07 94.78,18.07 C29.1
N$23
  Top 1.016: C11.1 129.35,32.52 129.35,33.78 129.75,34.18 R3.1
N$24  (via drill 0.35)
  Top 0.254: R9.2 85.38,30.38 v85.38,31.62 | v131.38,37.5 130.13,37.5 R3.2
  Bottom 0.254: v85.38,31.62 85.38,35.5 87.5,37.5 v131.38,37.5
  pour Top (no thermals): 129.75,43.5 120,43.5 120,33.62 128,33.62 128,35.75 129.75,35.75
N$25
  Top 1.016: C10.2 117.83,32.45 R5.1 121.02,32.28 D4.C
N$26  (via drill 0.35)
  Top 0.203: R28.1 69.44,9 70.19,9.75 v71.12,9.75 | v72.51,17.91 73.22,17.91 73.38,17.75 IC6.30
  Bottom 0.203: v72.51,17.91 71.25,16.65 71.25,9.88 v71.12,9.75
N$28
  pour Top: 65,52.12 75,52.12 75,41.62 75.12,41.5 65,41.5
N$31
  Top 0.254: R18.2 LED2.A
N$34
  Top 0.254: R17.2 LED1.A
N$35
  Top 0.203: LED4.C 129.18,25.07 129.18,21 127.77,19.59 K2.1
N$36
  Top 0.203: LED3.C 125.25,26.5 126.02,27.29 129.21,27.29 129.75,26.75 129.75,20.5 129.12,19.88 129.12,17.75 129.62,17.25 131.67,17.25 K1.1
NRST  (via drill 0.35)
  Top 0.254: C25.1 85.1,20.75 83.6,19.25 IC6.10 80.95,19.25 80.35,18.65 80.35,15.38 79.62,14.65 v79.62,14.5 | R27.1 78.53,1.43 v78.5,1.4 76.29,1.4 X5.10
  Bottom 0.254: v78.5,1.4 78.6,1.4 80.53,3.32 80.53,12.5 79.62,13.4 v79.62,14.5
OVP  (via drill 0.35)
  Top 0.203: R20.1 127.95,21.65 126.9,20.6 123.25,20.6 121.75,19.1 v121.75,18.5
  Top 0.254: v77.45,16.52 77.45,15.95 76.75,15.25 IC6.39
  Bottom 0.203: v77.45,16.52 83.05,16.52 83.99,15.58 90.41,15.58 91.17,16.35 119.6,16.35 v121.75,18.5
OVP_IN  (via drill 0.35)
  Top 0.203: K2.4 127.77,10.1 130,7.87 v130,2.38
  Bottom 0.203: X3.3 95.98,2.12 129.75,2.12 v130,2.38
OVP_OUT  (via drill 0.35)
  Top 0.203: v127.5,4.75 127.5,9.45 125.36,11.6 K2.3
  Bottom 0.203: v127.5,4.75 111.64,4.75 X4.3
R1  (via drill 0.35)
  Top 0.203: v77.9,11.8 78.25,12.15 IC6.42 | v78.5,3.74 78.34,3.9 X5.6
  Bottom 0.203: v78.5,3.74 77.74,4.5 77.74,11.64 v77.9,11.8
R2  (via drill 0.35)
  Top 0.203: IC6.37 74.7,13.25 v74.65,13.3
  Top 0.254: X5.8 78.47,2.63 v78.5,2.6
  Bottom 0.254: v74.65,13.3 74.65,12 74.9,11.75 74.9,6.2 v78.5,2.6
SWCLK
  Top 0.203: X5.4 74.83,5.17 74.25,5.75 74.25,7.38 72.38,9.25 72.38,10.9 R22.1 arc60 72.75,11.25 73.12,11.25 73.75,11.88 73.75,13.88 73.5,14.12 73.5,14.62 73.62,14.75 IC6.36
SWDIO  (via drill 0.35)
  Top 0.254: X5.2 76.25,6.57 73.25,9.62 v73.12,9.62 | IC6.35 v72.5,15.25
  Bottom 0.203: v73.12,9.62 73.12,14.38 72.5,15 v72.5,15.25
VCC  (via drill 0.35)
  Top 0.203: C34.1 80.67,10.9 IC8.3 78.92,10.75 78.34,10.75 77.84,10.25 IC8.5 | IC9.1 69.85,5.6 70.69,6.44 X5.1 72.35,7.3 v72.22,7.43
  Top 0.254: C24.1 90.58,21.5 | C28.1 85.33,18.95 v85.12,18.75 83.62,17.25 IC6.6 82.04,17.25 81.82,17.03 81.82,16.47 82.01,16.27 82.72,16.27 IC6.4 | IC7.7 107.83,18.9 | 107.83,18.9 107.83,18.68 108.5,18 114.2,18 115.44,19.25 IC7.1 | C27.1 104.47,18.9 107.83,18.9 | IC1.5 111.65,30.05 111.92,29.77 C15.1 | C34.1 80.72,11.05 81.97,12.3 v82.58,12.3 | v82.75,1.25 82.58,1.43 R27.2
  Top 0.305: C26.1 97.8,19.85 98.4,19.25 104.12,19.25 C27.1 | v90.45,23.45 91.85,23.45 v92.4,24 | C15.1 v110.72,28.6
  Top 0.61: 90.58,21.5 IC5.4 91.88,20.07 | 91.88,20.07 IC5.3 93.36,20.07 93.94,20.65 96.5,20.65 96.7,20.45 C26.1 97.8,22.05 IC4.5 | v90.45,23.45 90.62,23.27 C24.1 | 91.88,20.07 v91.88,18.27
  Route3 0.305: v105.8,24 106.15,24 110.72,28.57 v110.72,28.6
  Route3 0.406: v82.75,1.25 81.5,2.5 81.5,11.22 v82.58,12.3 81.97,12.9 77.35,12.9 v76.25,11.8
  Route3 0.61: v72.22,7.43 73.42,7.43 76.25,10.25 v76.25,11.8
  Bottom 0.254: v91.88,18.27 91.78,18.38 85.5,18.38 v85.12,18.75
  Bottom 0.305: v92.4,24 v105.8,24
  Bottom 0.61: v90.45,23.45 90.5,23.4 87.15,23.4 86.45,22.7 77.45,22.7 74.75,20 74.75,15.65 76.25,14.15 v76.25,11.8
VCC2  (via drill 0.35)
  Top 0.203: D6.C 122.07,11.25 122.25,11.25
  Top 0.254: 122.25,11.25 v122.25,9 115.38,2.12 109.19,2.12 X4.6 | IC7.16 117.53,11.4 C33.2 118.41,11.62 D6.C
  Route3 0.305: X6.6 125.81,9 v122.25,9 | X3.6 99.7,3.48 X4.6
VIN
  Top 0.203: R4.2 109,34.9 109.7,34.2 109.7,31.7 110.3,31.1 112.3,31.1 113.15,31.95 IC1.3 | 76.97,31.12 76.9,31.05 R8.1 R7.2
  Top 0.254: F1.2B 83.48,31.12 76.97,31.12
  Top 0.61: L1.1 89.15,27 C13.1 89.15,36.01 89.12,36.03 | F1.2B 83.7,36.03 | F1.2A 83.7,37.41 83.7,36.03 | 89.12,36.03 D3.C 95.25,36.03 C6.1 C8.1 C9.1 | 89.12,36.03 83.7,36.03
  pour Top (isolate 0.406, no thermals): 106.9,31.2 108.5,31.2 108.7,31.4 108.7,36.3 107.5,37.5 84.1,37.5 83.9,37.7 79.9,37.7 79.9,34.3 80.2,34 105.8,34 106.8,33 106.8,31.3
VREF  (via drill 0.35)
  Top 0.254: R24.1 78.85,6.6 77.75,7.7 v76.45,7.7 | v89.25,24.38 89.25,22.25 89.26,19.1 | C30.1 85.39,17.35 v85.14,17.61 84.28,16.75 IC6.5 | 89.26,19.1 89.26,18.2 | 89.26,18.2 v89.26,17.55 | IC5.6 89.28,18.18 89.26,18.2 | IC5.5 89.28,19.12 89.26,19.1 | R15.1 82.75,25.1 v82.75,23.62
  Bottom 0.254: v89.25,24.38 89,24.12 86.88,24.12 86.12,23.38 83,23.38 82.7,23.65 | 82.7,23.65 82.75,23.65 v82.75,23.62 | 82.7,23.65 77.28,23.65 74,20.38 74,15.41 75.5,13.91 75.5,8.65 v76.45,7.7 | v85.14,17.61 85.19,17.55 v89.26,17.55
VREF_
  Top 0.254: JP1.1 83.42,7.46 82.56,6.6 R24.2

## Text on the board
tPlace: ECS | - | + | www.ecs-online.org | ERROR | FUNC | LVP | OVP | IN | OUT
